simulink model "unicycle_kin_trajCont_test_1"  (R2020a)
settings: Solver=FixedStepAuto  StartTime=0.0  StopTime=inf  RelTol=1e-3
undefined symbols (not defined in the file or in its folder): desired_position, desired_velocity, geometry_msgs, Point, X, Y
libraries: robotlib x5

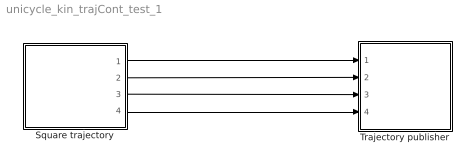
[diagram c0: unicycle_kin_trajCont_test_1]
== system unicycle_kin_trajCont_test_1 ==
  Square trajectory : Subsystem  mask{L=3, v=0.2, start=[0,0]}
      mask prompts: L "Side length"; v "Speed"; start "Start position [x, y]"
  Trajectory publisher : Subsystem  mask{simPublishRate=10}
      mask prompts: simPublishRate "Publising rate [Hz]"
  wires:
  Square trajectory/1(x) -> Trajectory publisher/1(xd)
  Square trajectory/2(y) -> Trajectory publisher/2(yd)
  Square trajectory/3(dx) -> Trajectory publisher/3(dxd)
  Square trajectory/4(dy) -> Trajectory publisher/4(dyd)

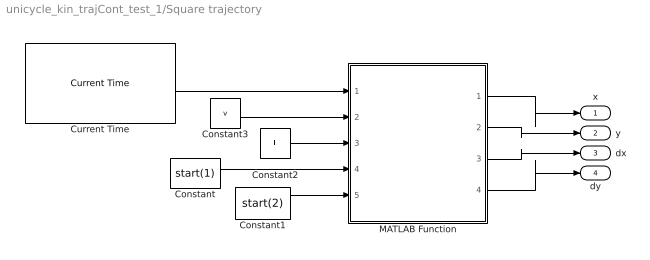
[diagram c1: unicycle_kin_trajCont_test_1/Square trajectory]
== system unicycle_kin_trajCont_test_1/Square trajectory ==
  Constant : Constant  Value=start(1)
  Constant1 : Constant  Value=start(2)
  Constant2 : Constant  Value=L
  Constant3 : Constant  Value=v
  Current Time : robotlib/Current Time  OutputFormat=double  SampleTime=-1  ModelName=unicycle_kin_trajCont_test
  MATLAB Function : MATLAB Function  TreatAsAtomicUnit=on
  x : Outport
  y : Outport  Port=2
  dx : Outport  Port=3
  dy : Outport  Port=4
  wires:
  MATLAB Function/2(y) -> y/1
  Constant3/1 -> MATLAB Function/2(v)
  Constant2/1 -> MATLAB Function/3(L)
  Constant1/1 -> MATLAB Function/5(y0)
  MATLAB Function/3(dx) -> dx/1
  MATLAB Function/4(dy) -> dy/1
  Current Time/1 -> MATLAB Function/1(t)
  Constant/1 -> MATLAB Function/4(x0)
  MATLAB Function/1(x) -> x/1

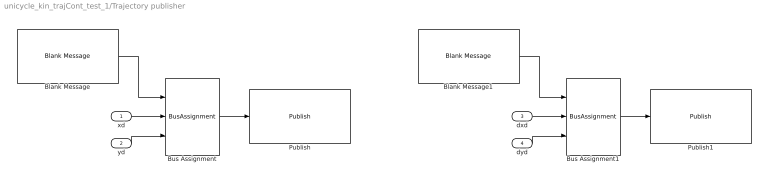
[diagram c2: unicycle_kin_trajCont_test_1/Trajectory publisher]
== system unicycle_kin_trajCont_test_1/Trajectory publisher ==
  xd : Inport  SampleTime=1/simPublishRate
  yd : Inport  Port=2  SampleTime=1/simPublishRate
  dxd : Inport  Port=3  SampleTime=1/simPublishRate
  dyd : Inport  Port=4  SampleTime=1/simPublishRate
  Blank Message : robotlib/Blank Message  messageClass=Message  entityType=geometry_msgs/Point  messageType=geometry_msgs/Point  SampleTime=1/simPublishRate
  Blank Message1 : robotlib/Blank Message  messageClass=Message  entityType=geometry_msgs/Point  messageType=geometry_msgs/Point  SampleTime=1/simPublishRate
  Bus Assignment : BusAssignment  AssignedSignals=X,Y
  Bus Assignment1 : BusAssignment  AssignedSignals=X,Y
  Publish : robotlib/Publish  topicSource=Specify your own  topic=/desired_position  messageType=geometry_msgs/Point  messageQueueLength=1
  Publish1 : robotlib/Publish  topicSource=Specify your own  topic=/desired_velocity  messageType=geometry_msgs/Point  messageQueueLength=1
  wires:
  Bus Assignment/1 -> Publish/1
  Blank Message/1 -> Bus Assignment/1
  xd/1 -> Bus Assignment/2
  yd/1 -> Bus Assignment/3
  dyd/1 -> Bus Assignment1/3
  dxd/1 -> Bus Assignment1/2
  Blank Message1/1 -> Bus Assignment1/1
  Bus Assignment1/1 -> Publish1/1

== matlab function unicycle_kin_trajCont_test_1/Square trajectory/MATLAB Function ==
function [x,y,dx,dy] = square_trajectory(t,v,L,x0,y0)

if (t<=L/v)
    x = x0+v*t;
    y = y0;
    dx = v;
    dy = 0;
elseif (t>L/v) && (t<=2*L/v)
    x = x0+L;
    y = y0+v*(t-L/v);
    dx = 0;
    dy = v;
elseif (t>2*L/v) && (t<=3*L/v)
    x = x0+L-v*(t-2*L/v);
    y = y0+L;
    dx = -v;
    dy = 0;
elseif (t>3*L/v) && (t<=4*L/v)
    x = x0;
    y = y0+L-v*(t-3*L/v);
    dx = 0;
    dy = -v;
else
    x = x0;
    y = y0;
    dx = 0;
    dy = 0;
end
